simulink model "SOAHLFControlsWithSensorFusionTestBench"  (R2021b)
settings: Solver=ode23tb  StartTime=0.0  StopTime=scenario.StopTime  RelTol=1e-3
PostLoadFcn:
  | helperSLHLFControlsWithSensorFusionSetup("testBenchModel","SOAHLFControlsWithSensorFusionTestBench")
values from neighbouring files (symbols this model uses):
  vehSim3D = repmat(     struct(         'Length', 0,         'RearOverhang', 0,         'InitialPos',[0 0 0],         'InitialRot',[0 0 0]),     numVehicles,1)    [helperSLHLFControlsWithSensorFusionSetup.m]
undefined symbols (not defined in the file or in its folder): actorProfiles, assessment, camera, m, n, scenario, Ts, v_set
libraries: drivingscenarioandsensors x8, sim3dautolib x6, simulink x4, sim3dprobsensorlib x1, sim3dlib x1, drivingsim3d x1

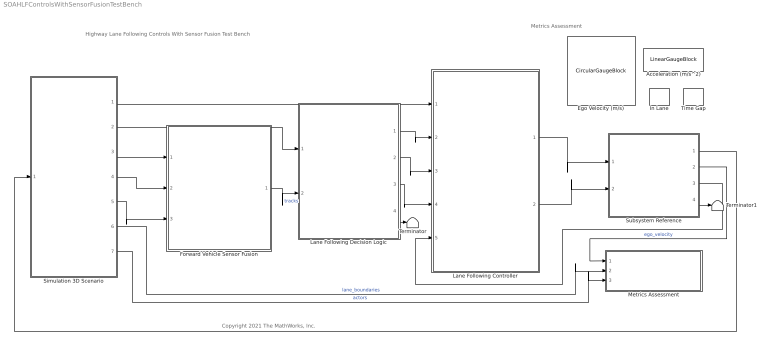
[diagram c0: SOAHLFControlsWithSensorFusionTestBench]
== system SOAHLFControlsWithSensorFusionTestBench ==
  note: Highway Lane Following Controls With Sensor Fusion Test Bench
  note: Metrics Assessment
  note: Copyright 2021 The MathWorks, Inc.
  Acceleration (m/s^2) : LinearGaugeBlock  LabelPosition=Hide  ScaleMin=-6  ScaleMax=6
  Ego Velocity (m/s) : CircularGaugeBlock  LabelPosition=Hide  ScaleMax=50
  Forward Vehicle Sensor Fusion : ModelReference  InputPortMessageModes=m,m,m  OutputPortMessageModes=m  ModelNameDialog=SOAForwardVehicleSensorFusion.slx  SimulationMode=Normal  CodeInterface=Top model  ModelReferenceVersion=5.17
  In Lane : LampBlock  LabelPosition=Hide
  Lane Following Controller : ModelReference  InputPortMessageModes=m,m,m,m,m  OutputPortMessageModes=m,m  ModelNameDialog=SOALaneFollowingController.slx  SimulationMode=Normal  ModelReferenceVersion=2.30
  Lane Following Decision Logic : ModelReference  InputPortMessageModes=m,m  OutputPortMessageModes=m,m,m,n  ModelNameDialog=SOALaneFollowingDecisionLogic.slx  SimulationMode=Normal  ModelReferenceVersion=2.22
  Metrics Assessment : Subsystem
  Simulation 3D Scenario : Subsystem  VariantControl=1
  Subsystem Reference : Subsystem  ReferencedSubsystem=SOAVehicleDynamics
  Terminator : Terminator
  Terminator1 : Terminator
  Time Gap : LampBlock  LabelPosition=Hide
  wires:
  Subsystem Reference/2 -> Metrics Assessment/1(Longitudinal Velocity)  "ego_velocity"
  Simulation 3D Scenario/3(System Time) -> Forward Vehicle Sensor Fusion/1
  Subsystem Reference/1 -> Simulation 3D Scenario/1(Ego)
  Simulation 3D Scenario/6(Lane Boundaries) -> Metrics Assessment/2(Lane Boundaries1)  "lane_boundaries"
  Simulation 3D Scenario/7(Actors) -> Metrics Assessment/3(Actors)  "actors"
  Lane Following Controller/1 -> Subsystem Reference/1
  Lane Following Controller/2 -> Subsystem Reference/2
  Simulation 3D Scenario/1(Set Velocity) -> Lane Following Controller/1
  Lane Following Decision Logic/1 -> Lane Following Controller/2
  Lane Following Decision Logic/3 -> Lane Following Controller/4
  Lane Following Decision Logic/2 -> Lane Following Controller/3
  Simulation 3D Scenario/4(Vision Detections) -> Forward Vehicle Sensor Fusion/2
  Simulation 3D Scenario/5(Radar Detections) -> Forward Vehicle Sensor Fusion/3
  Forward Vehicle Sensor Fusion/1 -> Lane Following Decision Logic/2  "tracks"
  Simulation 3D Scenario/2(Lanes) -> Lane Following Decision Logic/1
  Lane Following Decision Logic/4 -> Terminator/1
  Subsystem Reference/3 -> Lane Following Controller/5
  Subsystem Reference/4 -> Terminator1/1

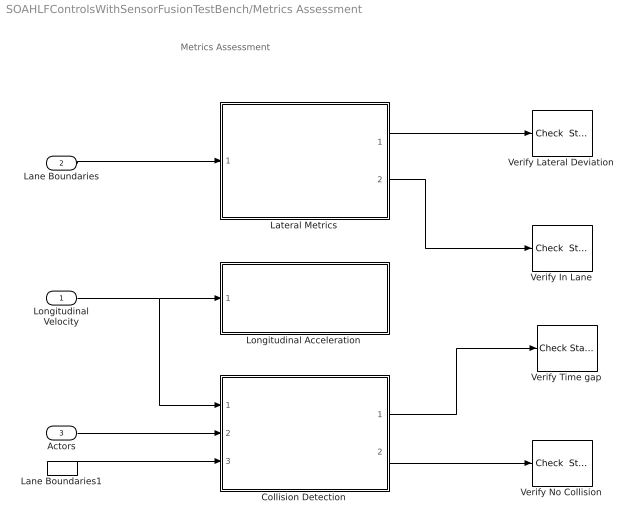
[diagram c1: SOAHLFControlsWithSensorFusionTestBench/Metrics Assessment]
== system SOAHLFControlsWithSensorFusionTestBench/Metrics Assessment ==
  note: Metrics Assessment
  Longitudinal Velocity : Inport
  Lane Boundaries : Inport  Port=2
  Actors : Inport  Port=3
  Collision Detection : Subsystem
  Lane Boundaries1 : InportShadow  Port=2
  Lateral Metrics : Subsystem
  Longitudinal Acceleration : Subsystem
  Verify In Lane : simulink/Model Verification/Check  Static Range  Description=1 <= u <= 1  max=1  max_included=on  min=1  min_included=on  enabled=on  stopWhenAssertionFail=on  export=off  icon=graphic
  Verify Lateral Deviation : simulink/Model Verification/Check  Static Range  Description=-assessment.LateralDeviationMax <= u <= assessment.LateralDeviationMax  max=assessment.LateralDeviationMax  max_included=on  min=-assessment.LateralDeviationMax  min_included=on  enabled=on  stopWhenAssertionFail=on  export=off  icon=graphic
  Verify No Collision : simulink/Model Verification/Check  Static Range  Description=0 <= u <= 0  max=0  max_included=on  min=0  min_included=on  enabled=on  stopWhenAssertionFail=on  export=off  icon=graphic
  Verify Time gap : simulink/Model Verification/Check Static  Lower Bound  Description=assessment.TimeGap <= u  min=assessment.TimeGap  min_included=on  enabled=on  stopWhenAssertionFail=off  export=off  icon=graphic
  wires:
  Actors/1 -> Collision Detection/2(Actors1)
  Lateral Metrics/1(Lateral Deviation) -> Verify Lateral Deviation/1
  Collision Detection/1(Time Gap) -> Verify Time gap/1
  Collision Detection/2(Collision) -> Verify No Collision/1
  Longitudinal Velocity/1 -> Collision Detection/1(Ego Velocity), Longitudinal Acceleration/1(Longitudinal Velocity)
  Lane Boundaries/1 -> Lateral Metrics/1(Lane Boundaries)
  Lane Boundaries1/1 -> Collision Detection/3(Lane Boundaries)
  Lateral Metrics/2(In Lane) -> Verify In Lane/1

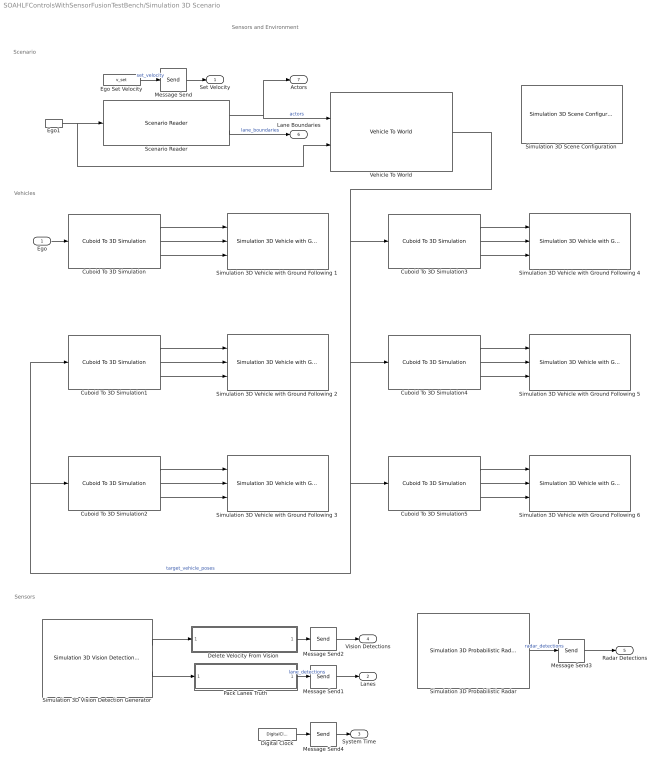
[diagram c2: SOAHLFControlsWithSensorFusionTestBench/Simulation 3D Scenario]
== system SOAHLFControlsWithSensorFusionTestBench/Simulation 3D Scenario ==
  note: Scenario
  note: Vehicles
  note: Sensors and Environment
  note: Sensors
  Ego : Inport
  Cuboid To 3D Simulation : drivingscenarioandsensors/Cuboid To 3D Simulation  SpecifyActorID=off  ActorIDToConvert=1  SimulateUsing=Interpreted execution
  Cuboid To 3D Simulation1 : drivingscenarioandsensors/Cuboid To 3D Simulation  SpecifyActorID=on  ActorIDToConvert=2  SimulateUsing=Interpreted execution
  Cuboid To 3D Simulation2 : drivingscenarioandsensors/Cuboid To 3D Simulation  SpecifyActorID=on  ActorIDToConvert=3  SimulateUsing=Interpreted execution
  Cuboid To 3D Simulation3 : drivingscenarioandsensors/Cuboid To 3D Simulation  SpecifyActorID=on  ActorIDToConvert=4  SimulateUsing=Interpreted execution
  Cuboid To 3D Simulation4 : drivingscenarioandsensors/Cuboid To 3D Simulation  SpecifyActorID=on  ActorIDToConvert=5  SimulateUsing=Interpreted execution
  Cuboid To 3D Simulation5 : drivingscenarioandsensors/Cuboid To 3D Simulation  SpecifyActorID=on  ActorIDToConvert=6  SimulateUsing=Interpreted execution
  "Delete Velocity From Vision " : MATLAB Function  TreatAsAtomicUnit=on  mask(Pack vision detections){structInit=Simulink.Bus.createMATLABStruct('BusVision'), measurementNoise=camera.MeasurementNoise}
      mask prompts: structInit "Output struct"; measurementNoise "Measurement noise"
      mask help: Packs vision detections to match bus used by vision processing algorithm. This includes replacing the measurement noise and disabling the velocity measurement.
  Digital Clock : DigitalClock  SampleTime=Ts
  Ego Set Velocity : Constant  Value=v_set  SampleTime=Ts
  Ego1 : InportShadow
  Message Send{,1..4} (5 alike) : Send  OutputPortMessageModes=m
  Pack Lanes Truth : MATLAB Function  TreatAsAtomicUnit=on  mask{structObj=Simulink.Bus.createMATLABStruct('LaneSensor')}
      mask prompts: structObj "Output struct"
  Scenario Reader : drivingscenarioandsensors/Scenario Reader  ScenarioSource=From workspace  ScenarioFileName=dblLaneChangeDrivingScenario.mat  ScenarioVariableName=scenario  OutputCoordinateSystem=Vehicle coordinates  EgoVehicleSource=Input port  EgoVehicleActorID=1  OrientVehiclesOnRoad=off  OutputEgoVehiclePose=off  OutputEgoVehicleState=off  SampleTime=0.1  LaneBoundaryOutput=Ego vehicle lane boundaries  LaneBoundaryDistance=0:0.5:70  LaneBoundaryLocation=Center of lane markings  BusNameSource=Auto  BusName=BusActors  BusNumActorsSource=Scenario  BusNumActors=100  BusName2Source=Auto  BusName2=BusLaneBoundaries  BusNumLaneBoundariesSource=Scenario  BusNumLaneBoundaries=10  BusName3Source=Auto  BusName3=BusEgoActor  BusName4Source=Auto  BusName4=BusEgoState  ShowCoordinateLabels=on  SimulateUsing=Interpreted execution
  Simulation 3D Probabilistic Radar : sim3dprobsensorlib/Simulation 3D Probabilistic Radar  Priority=1  sensorTag=Sim3dSensor2  sensorId=2  sensorName=Sim3dSensor2  vehTagList={'Scene Origin';'SimulinkVehicle1';'SimulinkVehicle4';'SimulinkVehicle5';'SimulinkVehicle6';'vehSim3D(2).InitialRot';'vehSim3D(3).InitialRot'}  vehTag=SimulinkVehicle1  mountLoc=Origin  offsetFlag=on  tmountOffset=radar.PositionSim3d  rmountOffset=radar.Rotation  AzimuthResolution=0.8  ElevationResolution=8  RangeResolution=1  RangeRateResolution=1  AzimuthBiasFraction=0.1  ElevationBiasFraction=0.1  RangeBiasFraction=0.05  RangeRateBiasFraction=0.05  FieldOfView=radar.FieldOfView  DetectionRange=radar.DetectionRanges  RangeRateLimits=[ -100, 100 ]  DetectionProbability=0.9  FalseAlarmRate=1e-6  ReferenceRange=150  ReferenceRCS=0  HasElevation=off  HasRangeRate=on  HasNoise=off  HasFalseAlarms=off  InitialSeedSource=Repeatable  InitialSeed=0  MaxNumDetections=50  DetectionCoordinates=Sensor spherical  SpecifyOutputBusName=off  BusName=BusSimulation3DRadarTruthSensor  SampleTime=-1  mountPoint=[2.424 0 0.8]  mountOrientation=[0 0 0]  aMode=3  ID=2
  Simulation 3D Scene Configuration : sim3dlib/Simulation 3D Scene Configuration  Priority=0  ProjectFormat_internal=Default Scenes  ProjectFormat=Default Scenes  SceneDesc=Curved road  ProjectName=/mathworks/devel/bat/BR2021bd/build/matlab/toolbox/shared/sim3d_projects/automotive_project/UE4/LinuxNoEditor/AutoVrtlEnv.sh  ScenePath=/Game/Maps/HwStrght  vehTagList={'Scene Origin';'SimulinkVehicle1';'SimulinkVehicle4';'SimulinkVehicle5';'SimulinkVehicle6';'vehSim3D(2).InitialRot';'vehSim3D(3).InitialRot'}  vehTag=SimulinkVehicle1  OpVisEn=off  Ts=0.1  EnableWindow=on  EnableWeather=off  SunAltitude=40.0  SunAzimuth=90  clouds=10  wind=1  fog=0  rain=0  sensorTag=MainCamera1  sensorId=1  sensorName=MainCamera1  mountLoc=Origin  offsetFlag=off  tmountOffset=[0, 0, 0]  rmountOffset=[0, 0, 0]  HorizontalResolution=1280  VerticalResolution=720  HorizontalFOV=60  mountPoint=[0 0 0]  mountOrientation=[0 0 0]  aMode=3  ID=1
  Simulation 3D Vehicle with Ground Following 1 : sim3dautolib/Simulation 3D Vehicle with Ground Following  Priority=-1  PassVehMesh=Sedan  PassVehMesh_Internal=Sedan  MeshPath=/MathWorksSimulation/Vehicles/Muscle/Meshes/SK_MuscleCar.SK_MuscleCar  TrackWidth=1.9  WheelBase=3  WheelRadius=0.35  VehColor=Blue  VehColor_Internal=Blue  InitialPos=vehSim3D(1).InitialPos  InitialRot=vehSim3D(1).InitialRot  ActorName=SimulinkVehicle1  SampleTime=-1  ActorType=SimulinkVehicle  ID=1  aMode=3  ActorTag=SimulinkVehicle1  CoordinateScheme=ISO  VehLightsControl=off  HeadlightColor=[ 1, 1, 1 ]  HighBeamIntensity=100000  LowBeamIntensity=60000  HighBeamConeAngle=70  LowBeamConeAngle=70  LeftHeadlightOrientation=[ 0, 0 ]  RightHeadlightOrientation=[ 0, 0 ]  BrakelightIntensity=500  ReverselightIntensity=500  SignallightIntensity=500  SignallightPeriod=1  SignalPulseWidth=50  TransformOutportEnabled=off
  Simulation 3D Vehicle with Ground Following 2 : sim3dautolib/Simulation 3D Vehicle with Ground Following  Priority=-1  PassVehMesh=Sedan  PassVehMesh_Internal=Sedan  MeshPath=/MathWorksSimulation/Vehicles/Muscle/Meshes/SK_MuscleCar.SK_MuscleCar  TrackWidth=1.9  WheelBase=3  WheelRadius=0.35  VehColor=Red  VehColor_Internal=Red  InitialPos=vehSim3D(2).InitialPos  InitialRot=vehSim3D(2).InitialRot  ActorName=vehSim3D(2).InitialRot  SampleTime=-1  ActorType=SimulinkVehicle  ID=C  aMode=3  ActorTag=vehSim3D(2).InitialRot  CoordinateScheme=ISO  VehLightsControl=off  HeadlightColor=[ 1, 1, 1 ]  HighBeamIntensity=100000  LowBeamIntensity=60000  HighBeamConeAngle=70  LowBeamConeAngle=70  LeftHeadlightOrientation=[ 0, 0 ]  RightHeadlightOrientation=[ 0, 0 ]  BrakelightIntensity=500  ReverselightIntensity=500  SignallightIntensity=500  SignallightPeriod=1  SignalPulseWidth=50  TransformOutportEnabled=off
  Simulation 3D Vehicle with Ground Following 3 : sim3dautolib/Simulation 3D Vehicle with Ground Following  Priority=-1  PassVehMesh=Muscle car  PassVehMesh_Internal=Muscle car  MeshPath=/MathWorksSimulation/Vehicles/Muscle/Meshes/SK_MuscleCar.SK_MuscleCar  TrackWidth=1.9  WheelBase=3  WheelRadius=0.35  VehColor=Black  VehColor_Internal=Black  InitialPos=vehSim3D(3).InitialPos  InitialRot=vehSim3D(3).InitialRot  ActorName=vehSim3D(3).InitialRot  SampleTime=-1  ActorType=SimulinkVehicle  ID=C  aMode=3  ActorTag=vehSim3D(3).InitialRot  CoordinateScheme=ISO  VehLightsControl=off  HeadlightColor=[ 1, 1, 1 ]  HighBeamIntensity=100000  LowBeamIntensity=60000  HighBeamConeAngle=70  LowBeamConeAngle=70  LeftHeadlightOrientation=[ 0, 0 ]  RightHeadlightOrientation=[ 0, 0 ]  BrakelightIntensity=500  ReverselightIntensity=500  SignallightIntensity=500  SignallightPeriod=1  SignalPulseWidth=50  TransformOutportEnabled=off
  Simulation 3D Vehicle with Ground Following 4 : sim3dautolib/Simulation 3D Vehicle with Ground Following  Priority=-1  PassVehMesh=Hatchback  PassVehMesh_Internal=Hatchback  MeshPath=/MathWorksSimulation/Vehicles/Muscle/Meshes/SK_MuscleCar.SK_MuscleCar  TrackWidth=1.9  WheelBase=3  WheelRadius=0.35  VehColor=Orange  VehColor_Internal=Orange  InitialPos=vehSim3D(4).InitialPos  InitialRot=vehSim3D(4).InitialRot  ActorName=SimulinkVehicle4  SampleTime=-1  ActorType=SimulinkVehicle  ID=4  aMode=3  ActorTag=SimulinkVehicle4  CoordinateScheme=ISO  VehLightsControl=off  HeadlightColor=[ 1, 1, 1 ]  HighBeamIntensity=100000  LowBeamIntensity=60000  HighBeamConeAngle=70  LowBeamConeAngle=70  LeftHeadlightOrientation=[ 0, 0 ]  RightHeadlightOrientation=[ 0, 0 ]  BrakelightIntensity=500  ReverselightIntensity=500  SignallightIntensity=500  SignallightPeriod=1  SignalPulseWidth=50  TransformOutportEnabled=off
  Simulation 3D Vehicle with Ground Following 5 : sim3dautolib/Simulation 3D Vehicle with Ground Following  Priority=-1  PassVehMesh=Small pickup truck  PassVehMesh_Internal=Small pickup truck  MeshPath=/MathWorksSimulation/Vehicles/Muscle/Meshes/SK_MuscleCar.SK_MuscleCar  TrackWidth=1.9  WheelBase=3  WheelRadius=0.35  VehColor=Green  VehColor_Internal=Green  InitialPos=vehSim3D(5).InitialPos  InitialRot=vehSim3D(5).InitialRot  ActorName=SimulinkVehicle5  SampleTime=-1  ActorType=SimulinkVehicle  ID=5  aMode=3  ActorTag=SimulinkVehicle5  CoordinateScheme=ISO  VehLightsControl=off  HeadlightColor=[ 1, 1, 1 ]  HighBeamIntensity=100000  LowBeamIntensity=60000  HighBeamConeAngle=70  LowBeamConeAngle=70  LeftHeadlightOrientation=[ 0, 0 ]  RightHeadlightOrientation=[ 0, 0 ]  BrakelightIntensity=500  ReverselightIntensity=500  SignallightIntensity=500  SignallightPeriod=1  SignalPulseWidth=50  TransformOutportEnabled=off
  Simulation 3D Vehicle with Ground Following 6 : sim3dautolib/Simulation 3D Vehicle with Ground Following  Priority=-1  PassVehMesh=Sport utility vehicle  PassVehMesh_Internal=Sport utility vehicle  MeshPath=/MathWorksSimulation/Vehicles/Muscle/Meshes/SK_MuscleCar.SK_MuscleCar  TrackWidth=1.9  WheelBase=3  WheelRadius=0.35  VehColor=Blue  VehColor_Internal=Blue  InitialPos=vehSim3D(6).InitialPos  InitialRot=vehSim3D(6).InitialRot  ActorName=SimulinkVehicle6  SampleTime=-1  ActorType=SimulinkVehicle  ID=6  aMode=3  ActorTag=SimulinkVehicle6  CoordinateScheme=ISO  VehLightsControl=off  HeadlightColor=[ 1, 1, 1 ]  HighBeamIntensity=100000  LowBeamIntensity=60000  HighBeamConeAngle=70  LowBeamConeAngle=70  LeftHeadlightOrientation=[ 0, 0 ]  RightHeadlightOrientation=[ 0, 0 ]  BrakelightIntensity=500  ReverselightIntensity=500  SignallightIntensity=500  SignallightPeriod=1  SignalPulseWidth=50  TransformOutportEnabled=off
  Simulation 3D Vision Detection Generator : drivingsim3d/Simulation 3D Vision Detection Generator  Priority=1  sensorTag=Sim3dSensor255  sensorId=1  sensorName=Sim3dSensor1  vehTagList={'Scene Origin';'SimulinkVehicle1';'SimulinkVehicle4';'SimulinkVehicle5';'SimulinkVehicle6';'vehSim3D(2).InitialRot';'vehSim3D(3).InitialRot'}  vehTag=SimulinkVehicle1  mountLoc=Origin  offsetFlag=on  tmountOffset=camera.PositionSim3d  rmountOffset=camera.Rotation  DetectorOutput=Objects only  MaxNumDetections=20  MaxNumLanes=30  laneSampleDistances=0:0.5:9.5  BusNameSource=Property  BusName=BusObjectDetections  BusName2Source=Property  BusName2=BusLaneDetections  MaxRange=camera.DetectionRanges(2)  BoundingBoxAccuracy=5  ProcessNoiseIntensity=5  MaxSpeed=50  MaxAllowedOcclusion=0.5  MinObjectImageSize=camera.MinObjectImageSize  DetectionProbability=1  FalsePositivesPerImage=0  MinLaneImageSize=[ 20, 3 ]  LaneBoundaryAccuracy=3  HasNoise=off  InitialSeedSource=Repeatable  InitialSeed=1  uniqueActorIdentifier=[]  actorClassInteger=0  cuboidLength=4.7  cuboidWidth=1.8  cuboidHeight=1.4  rotationalCenter={[-1.35, 0, 0]}  focalLength=camera.FocalLength  opticalCenter=camera.PrincipalPoint  imageSize=camera.ImageSize  radialDistortionCoefficients=[0, 0]  tangentialDistortionCoefficients=[0, 0]  cameraAxisSkew=0  actorTruthOutportEnabled=off  laneTruthOutportEnabled=on  SampleTime=-1  checkedSampleTime=0.1  mountPoint=[0.57 0 1.2]  mountOrientation=[0 0 0]  aMode=3  ID=1
  Vehicle To World : drivingscenarioandsensors/Vehicle To World  BusNameSource=Auto  BusName=BusVehicleToWorldActors  SimulateUsing=Interpreted execution
  Set Velocity : Outport  Unit=m/s  VectorParamsAs1DForOutWhenUnconnected=off
  Lanes : Outport  Port=2
  System Time : Outport  Port=3  VectorParamsAs1DForOutWhenUnconnected=off
  Vision Detections : Outport  Port=4
  Radar Detections : Outport  Port=5
  Lane Boundaries : Outport  Port=6
  Actors : Outport  Port=7
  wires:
  Cuboid To 3D Simulation/2 -> Simulation 3D Vehicle with Ground Following 1/2
  Cuboid To 3D Simulation/1 -> Simulation 3D Vehicle with Ground Following 1/1
  Cuboid To 3D Simulation/3 -> Simulation 3D Vehicle with Ground Following 1/3
  Ego/1 -> Cuboid To 3D Simulation/1
  Cuboid To 3D Simulation1/2 -> Simulation 3D Vehicle with Ground Following 2/2
  Cuboid To 3D Simulation1/1 -> Simulation 3D Vehicle with Ground Following 2/1
  Cuboid To 3D Simulation1/3 -> Simulation 3D Vehicle with Ground Following 2/3
  Scenario Reader/1 -> Vehicle To World/1, Actors/1  "actors"
  Vehicle To World/1 -> Cuboid To 3D Simulation3/1, Cuboid To 3D Simulation4/1, Cuboid To 3D Simulation5/1, Cuboid To 3D Simulation2/1, Cuboid To 3D Simulation1/1  "target_vehicle_poses"
  Cuboid To 3D Simulation3/2 -> Simulation 3D Vehicle with Ground Following 4/2
  Cuboid To 3D Simulation3/3 -> Simulation 3D Vehicle with Ground Following 4/3
  Cuboid To 3D Simulation2/2 -> Simulation 3D Vehicle with Ground Following 3/2
  Cuboid To 3D Simulation3/1 -> Simulation 3D Vehicle with Ground Following 4/1
  Cuboid To 3D Simulation2/3 -> Simulation 3D Vehicle with Ground Following 3/3
  Cuboid To 3D Simulation2/1 -> Simulation 3D Vehicle with Ground Following 3/1
  Cuboid To 3D Simulation4/3 -> Simulation 3D Vehicle with Ground Following 5/3
  Cuboid To 3D Simulation5/2 -> Simulation 3D Vehicle with Ground Following 6/2
  Cuboid To 3D Simulation5/3 -> Simulation 3D Vehicle with Ground Following 6/3
  Cuboid To 3D Simulation5/1 -> Simulation 3D Vehicle with Ground Following 6/1
  Cuboid To 3D Simulation4/2 -> Simulation 3D Vehicle with Ground Following 5/2
  Cuboid To 3D Simulation4/1 -> Simulation 3D Vehicle with Ground Following 5/1
  Scenario Reader/2 -> Lane Boundaries/1  "lane_boundaries"
  Ego1/1 -> Vehicle To World/2, Scenario Reader/1
  Ego Set Velocity/1 -> Message Send/1  "set_velocity"
  Simulation 3D Vision Detection Generator/1 -> "Delete Velocity From Vision "/1(detections)
  Simulation 3D Probabilistic Radar/1 -> Message Send3/1  "radar_detections"
  "Delete Velocity From Vision "/1(updatedDetections) -> Message Send2/1
  Digital Clock/1 -> Message Send4/1
  Simulation 3D Vision Detection Generator/2 -> Pack Lanes Truth/1(lanesTruth)
  Pack Lanes Truth/1(lanes) -> Message Send1/1  "lane_detections"
  Message Send/1 -> Set Velocity/1
  Message Send1/1 -> Lanes/1
  Message Send3/1 -> Radar Detections/1
  Message Send2/1 -> Vision Detections/1
  Message Send4/1 -> System Time/1

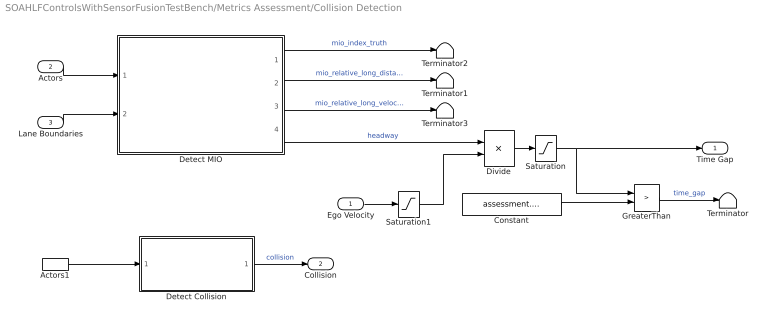
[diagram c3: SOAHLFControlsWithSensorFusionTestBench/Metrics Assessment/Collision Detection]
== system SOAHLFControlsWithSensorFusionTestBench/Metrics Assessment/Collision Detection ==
  Ego Velocity : Inport
  Actors : Inport  Port=2
  Lane Boundaries : Inport  Port=3
  Actors1 : InportShadow  Port=2
  Constant : Constant  Value=assessment.TimeGap
  Detect Collision : MATLAB Function  TreatAsAtomicUnit=on  mask(Detect Collision){vehicleProfiles=actorProfiles(scenario)}
      mask prompts: vehicleProfiles "Vehicle profiles"
      mask help: Detect collision between ego and target vehicles. Vehicle profiles is expected to be the struture returned by the actorProfiles method of a drivingScenerio object.
  Detect MIO : MATLAB Function  TreatAsAtomicUnit=on  mask(Detect Most Important Obejct (MIO)){vehicleProfiles=actorProfiles(scenario)}
      mask prompts: vehicleProfiles "Vehicle profiles"
      mask help: Detect most important object (MIO) in ego vehicle lane. Headway to MIO takes into account the vehicel dimensions. Vehicle profiles is expected to be the struture returned by the actorProfiles method of a drivingScenerio object.
  Divide : Product  Inputs=*/
  GreaterThan : RelationalOperator  Operator=>  OutDataTypeStr=boolean  RndMeth=Simplest
  Saturation : Saturate  UpperLimit=4  LowerLimit=0
  Saturation1 : Saturate  UpperLimit=100  LowerLimit=0.01
  Terminator{,1..3} (4 alike) : Terminator
  Time Gap : Outport
  Collision : Outport  Port=2
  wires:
  Actors/1 -> Detect MIO/1(actors)
  Lane Boundaries/1 -> Detect MIO/2(lane)
  Detect MIO/4(headway) -> Divide/1  "headway"
  Ego Velocity/1 -> Saturation1/1
  Divide/1 -> Saturation/1
  Saturation/1 -> Time Gap/1, GreaterThan/1
  Saturation1/1 -> Divide/2
  Constant/1 -> GreaterThan/2
  GreaterThan/1 -> Terminator/1  "time_gap"
  Detect MIO/2(mioRelLongDist) -> Terminator1/1  "mio_relative_long_distance_truth"
  Detect MIO/1(mioIndex) -> Terminator2/1  "mio_index_truth"
  Detect Collision/1(collision) -> Collision/1  "collision"
  Detect MIO/3(mioRelLongVel) -> Terminator3/1  "mio_relative_long_velocity_truth"
  Actors1/1 -> Detect Collision/1(actors)

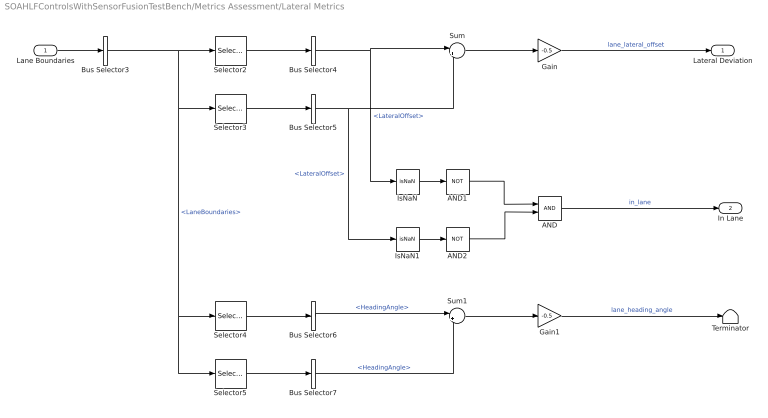
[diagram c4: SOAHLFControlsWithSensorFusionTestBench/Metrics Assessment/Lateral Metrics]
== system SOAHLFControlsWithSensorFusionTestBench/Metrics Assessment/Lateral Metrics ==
  Lane Boundaries : Inport
  AND : Logic  IconShape=distinctive  AllPortsSameDT=off  OutDataTypeStr=boolean
  AND1 : Logic  Operator=NOT  IconShape=distinctive  AllPortsSameDT=off  OutDataTypeStr=boolean
  AND2 : Logic  Operator=NOT  IconShape=distinctive  AllPortsSameDT=off  OutDataTypeStr=boolean
  Bus Selector3 : BusSelector  OutputSignals=LaneBoundaries
  Bus Selector4 : BusSelector  OutputSignals=LateralOffset
  Bus Selector5 : BusSelector  OutputSignals=LateralOffset
  Bus Selector6 : BusSelector  OutputSignals=HeadingAngle
  Bus Selector7 : BusSelector  OutputSignals=HeadingAngle
  Gain : Gain  Gain=-0.5
  Gain1 : Gain  Gain=-0.5
  IsNaN : RelationalOperator  Operator=isNaN  OutDataTypeStr=boolean  RndMeth=Simplest
  IsNaN1 : RelationalOperator  Operator=isNaN  OutDataTypeStr=boolean  RndMeth=Simplest
  Selector2 : Selector  InputPortWidth=2  IndexOptions=Index vector (dialog)  Indices=1  OutputSizes=1
  Selector3 : Selector  InputPortWidth=2  IndexOptions=Index vector (dialog)  Indices=2  OutputSizes=1
  Selector4 : Selector  InputPortWidth=2  IndexOptions=Index vector (dialog)  Indices=1  OutputSizes=1
  Selector5 : Selector  InputPortWidth=2  IndexOptions=Index vector (dialog)  Indices=2  OutputSizes=1
  Sum : Sum  Inputs=|++
  Sum1 : Sum  Inputs=|++
  Terminator : Terminator
  Lateral Deviation : Outport  VectorParamsAs1DForOutWhenUnconnected=off
  In Lane : Outport  Port=2
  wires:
  AND/1 -> In Lane/1  "in_lane"
  IsNaN1/1 -> AND2/1
  IsNaN/1 -> AND1/1
  Sum/1 -> Gain/1
  Bus Selector5/1 -> IsNaN1/1, Sum/2  "<LateralOffset>"
  Selector2/1 -> Bus Selector4/1
  Bus Selector4/1 -> IsNaN/1, Sum/1  "<LateralOffset>"
  Selector3/1 -> Bus Selector5/1
  Lane Boundaries/1 -> Bus Selector3/1
  Gain/1 -> Lateral Deviation/1  "lane_lateral_offset"
  AND1/1 -> AND/1
  AND2/1 -> AND/2
  Selector5/1 -> Bus Selector7/1
  Bus Selector6/1 -> Sum1/1  "<HeadingAngle>"
  Selector4/1 -> Bus Selector6/1
  Bus Selector3/1 -> Selector2/1, Selector3/1, Selector4/1, Selector5/1  "<LaneBoundaries>"
  Sum1/1 -> Gain1/1
  Bus Selector7/1 -> Sum1/2  "<HeadingAngle>"
  Gain1/1 -> Terminator/1  "lane_heading_angle"

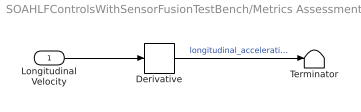
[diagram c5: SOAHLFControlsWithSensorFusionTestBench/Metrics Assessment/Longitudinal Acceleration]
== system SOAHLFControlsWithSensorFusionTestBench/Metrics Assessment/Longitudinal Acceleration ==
  Longitudinal Velocity : Inport
  Derivative : Derivative
  Terminator : Terminator
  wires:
  Derivative/1 -> Terminator/1  "longitudinal_acceleration"
  Longitudinal Velocity/1 -> Derivative/1

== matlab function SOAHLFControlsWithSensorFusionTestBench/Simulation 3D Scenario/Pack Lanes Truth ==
function lanes = packLanesTruth(lanesTruth, structObj)
% Assign lane parameters from ground-truth lane boundaries.

% Assign lanes struct object to output variable
lanes = structObj;

% Find ego-vehicle lane boundary indices
lbNum = [1, 1];
for j = 1:length(lanesTruth.LaneBoundaries)-1
    yleftLane = lanesTruth.LaneBoundaries(j+1).Coordinates(1,2);
    yrightLane = lanesTruth.LaneBoundaries(j).Coordinates(1,2);
    
    if ((0 >= yleftLane) && (0 <= yrightLane))
        lbNum(1) = j;
        lbNum(2) = j+1;
        break;
    elseif ((0 >= yrightLane) && (0 <= yleftLane))
        lbNum(1) = j+1;
        lbNum(2) = j;
        break;
    end
end

%% Pack left lane info
leftLaneCoordinates = lanesTruth.LaneBoundaries(lbNum(1)).Coordinates;
% Get parabolic lane boundary parameters using polyfit for the left lane.
leftLaneParameters = polyfit(leftLaneCoordinates(:,1),...
    leftLaneCoordinates(:,2),2);

% Assign lane parameters to output bus, lanes.
lanes.Left.Curvature = single(2 * leftLaneParameters(1));
lanes.Left.HeadingAngle = single(leftLaneParameters(2));
lanes.Left.LateralOffset = single(leftLaneParameters(3));

lanes.Left.Strength = single(lanesTruth.LaneBoundaries(lbNum(1)).Strength);


%% Pack right lane info
rightLaneCoordinates = lanesTruth.LaneBoundaries(lbNum(2)).Coordinates;
% Get parabolic lane boundary parameters using polyfit for the right lane
rightLaneParameters = polyfit(rightLaneCoordinates(:,1),...
    rightLaneCoordinates(:,2),2);

% Assign lane parameters to output bus, lanes.
lanes.Right.Curvature = single(2 * rightLaneParameters(1));
lanes.Right.HeadingAngle = single(rightLaneParameters(2));
lanes.Right.LateralOffset = single(rightLaneParameters(3));

lanes.Right.Strength = single(lanesTruth.LaneBoundaries(lbNum(2)).Strength);

end

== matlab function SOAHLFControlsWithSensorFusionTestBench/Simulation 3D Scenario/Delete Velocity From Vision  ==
function updatedDetections = deleteVelocityFromVision(detections,structInit,measurementNoise)

updatedDetections = structInit;
updatedDetections.NumDetections = detections.NumDetections;
updatedDetections.IsValidTime = detections.IsValidTime;
for n = 1:detections.NumDetections
    updatedDetections.Detections(n).Time = detections.Detections(n).Time;
    updatedDetections.Detections(n).Measurement = detections.Detections(n).Measurement(1:3);
    updatedDetections.Detections(n).MeasurementNoise = measurementNoise;
    updatedDetections.Detections(n).SensorIndex = detections.Detections(n).SensorIndex;
    updatedDetections.Detections(n).ObjectClassID = detections.Detections(n).ObjectClassID;
    updatedDetections.Detections(n).ObjectAttributes = detections.Detections(n).ObjectAttributes;
    updatedDetections.Detections(n).MeasurementParameters = detections.Detections(n).MeasurementParameters;
    updatedDetections.Detections(n).MeasurementParameters.HasVelocity = false;
end

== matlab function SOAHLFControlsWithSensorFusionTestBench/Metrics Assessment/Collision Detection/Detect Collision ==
function collision = detectCollision(actors, vehicleProfiles)

% Associate on-path MATLAB function
coder.extrinsic('helperSLDetectVehicleCollision');

% Assign default value to define output data type
collision = false;

% Call on-path MATLAB function
collision = helperSLDetectVehicleCollision(actors.Actors, vehicleProfiles);

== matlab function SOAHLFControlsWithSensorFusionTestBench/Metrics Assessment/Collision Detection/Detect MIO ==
function [mioIndex,mioRelLongDist,mioRelLongVel,headway] = detectMIO(actors,lane,vehicleProfiles)

% Find the closest vehicle in ego lane
longDist = zeros(1,actors.NumActors);
for i = 1:actors.NumActors
    
    % Positions with respect to ego
    x = actors.Actors(i).Position(1);
    y = actors.Actors(i).Position(2);
    
    % Default longitudinal distance from vehicle
    longDist(i) = inf;
    
    % Check if vehicle is ahead of ego
    if x >= 0
        % Find left lane coordinates closest to vehicle position x
        [~,n] = min(abs(lane.LaneBoundaries(1).Coordinates(:,1)-x));
        yleftLane = lane.LaneBoundaries(1).Coordinates(n,2);

        % Find right lane coordinates closest to vehicle position x
        [~,n] = min(abs(lane.LaneBoundaries(2).Coordinates(:,1)-x));
        yrightLane = lane.LaneBoundaries(2).Coordinates(n,2);

        % Check if vehicle is in same lane as ego
        if (yrightLane <= y) && (y <= yleftLane)
            longDist(i) = x;
        end       
    end
end

% Minimum distance between vehicle rear axles
[minLongDist,mioIndex] = min(longDist);

if isempty(minLongDist) || isinf(minLongDist)
    mioIndex = nan;
    mioRelLongDist = inf;
    mioRelLongVel = inf;
    headway = inf;
else
    mioRelLongDist = minLongDist;
    mioRelLongVel = actors.Actors(mioIndex).Velocity(1);
    headway = headwayLongDist(minLongDist,mioIndex,vehicleProfiles);
end

end

function headway = headwayLongDist(dist,mioIndex,vehicleProfiles)
% Longitudinal headway is distance between vehicle rear axles
% reduced by distance of ego rear axle to front and 
% reduced by distance of MIO rear axle to rear

% Notes on origin offset
% - Origin offset is the relative position [x,yz] of vehicle center with 
%   respect to the rear axle
% - Distance rear axle center to vehicle center = negative of origin offset(1)

% Ego distance from rear axle to front
egoProfile = vehicleProfiles(1);
egoDistRearAxleToVehCenter = - egoProfile.OriginOffset(1);
egoDistRearAxleToFront = egoProfile.Length/2 + egoDistRearAxleToVehCenter;

% MIO distance from rear axle to rear
mioProfile = vehicleProfiles(mioIndex);
mioDistRearAxleToVehCenter = - mioProfile.OriginOffset(1);
mioDistRearAxleToRear = mioProfile.Length/2 - mioDistRearAxleToVehCenter;

% Longitudinal headway is distance from front of ego to rear of MIO
headway = dist - egoDistRearAxleToFront - mioDistRearAxleToRear;

end
